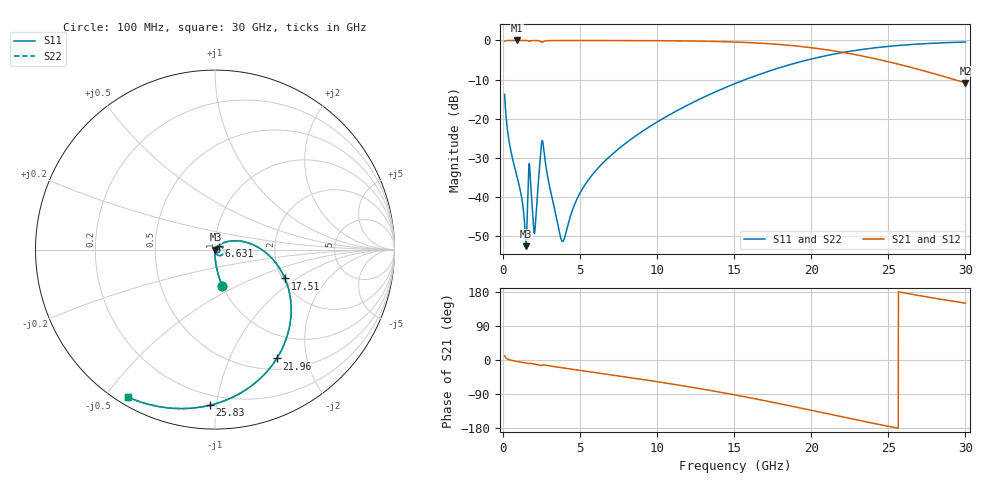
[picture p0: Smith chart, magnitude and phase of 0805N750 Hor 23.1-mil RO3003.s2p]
# GHz S MA R 50
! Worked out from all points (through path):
!   3201 points, 100 MHz to 30 GHz, reference 50 ohm
!   highest |S21| = -0.01 dB at 912.9 MHz (marker M1); lowest = -10.8 dB at 30 GHz (marker M2)
!   group delay of S21, straight-line fit = 20.3 ps
!   lowest |S11| = -52.5 dB at 1.492 GHz (marker M3), VSWR 1.00, Z = 50.2 - j0.0989 ohm
!   |S11| at or under -10 dB: start of sweep to 15.71 GHz
!   |S22| runs from -52.5 to -0.4 dB; largest |S21 - S12| = 0
!   S11 on the Smith chart (normalised r, x): 100 MHz: 1.00, -0.42; 6.631 GHz: 1.04, +0.05; 17.51 GHz: 2.06, -0.81; 21.96 GHz: 0.64, -1.52; 25.83 GHz: 0.14, -0.96; 30 GHz: 0.03, -0.57
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0.1  0.2052 -78.6  0.9784 11.3  0.9784 11.3  0.2052 -78.6
0.4270312  0.04711 -89.0  0.9984 0.4  0.9984 0.4  0.04711 -89.0
0.9129063  0.01811 -91.5  0.999 -3.9  0.999 -3.9  0.01811 -91.5
1.193219  0.01021 -90.3  0.9989 -5.8  0.9989 -5.8  0.01021 -90.3
1.398781  0.004571 -78.4  0.9985 -7.3  0.9985 -7.3  0.004571 -78.4
1.492219  0.002379 -24.4  0.9977 -8.0  0.9977 -8.0  0.002379 -24.4
1.735156  0.02311 -45.5  0.9814 -8.5  0.9814 -8.5  0.02311 -45.5
1.959406  0.00472 -52.5  0.9964 -10.3  0.9964 -10.3  0.00472 -52.5
2.080875  0.004064 15.1  0.9963 -11.3  0.9963 -11.3  0.004064 15.1
2.41725  0.03254 30.0  0.9764 -14.3  0.9764 -14.3  0.03254 30.0
2.557406  0.05239 -24.9  0.9486 -13.1  0.9486 -13.1  0.05239 -24.9
3.818812  0.002769 -25.8  0.9971 -20.4  0.9971 -20.4  0.002769 -25.8
5.089563  0.01224 50.6  0.9973 -27.8  0.9973 -27.8  0.01224 50.6
6.631281  0.02929 48.1  0.9967 -36.8  0.9967 -36.8  0.02929 48.1
10.06978  0.09299 30.3  0.992 -57.7  0.992 -57.7  0.09299 30.3
15.05  0.2816 -3.1  0.9542 -92.1  0.9542 -92.1  0.2816 -3.1
17.50741  0.4214 -22.4  0.9005 -111.7  0.9005 -111.7  0.4214 -22.4
20.03956  0.5819 -43.8  0.8059 -133.2  0.8059 -133.2  0.5819 -43.8
21.96438  0.6975 -60.4  0.7086 -149.9  0.7086 -149.9  0.6975 -60.4
25.01978  0.8401 -85.7  0.5334 -175.1  0.5334 -175.1  0.8401 -85.7
25.83269  0.8678 -91.9  0.4876 178.6  0.4876 178.6  0.8678 -91.9
30  0.9543 -120.5  0.2877 150.0  0.2877 150.0  0.9543 -120.5
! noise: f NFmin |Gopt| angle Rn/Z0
0.1  0.000449  0.8656  0.6637  0.0007176
3.417  0.008061  0.7603  18.31  0.006645
6.743  0.01008  0.6516  35.49  0.005015
10.06  0.01372  0.6318  51.71  0.005737
13.39  0.01788  0.6342  66.89  0.006545
16.7  0.02289  0.6507  81  0.007437
20.03  0.02932  0.6785  94.33  0.008493
23.35  0.03801  0.716  107.1  0.0098
26.67  0.05055  0.7619  119.7  0.01144
30  0.06986  0.813  132.5  0.01337
